(* Logix 5000 AddOnInstructionDefinition export AMP_Relative_Move; software revision 20.04 *)

TYPE AMP_Status_Word :   // Applied Motion Input Assembly Status Word
STRUCT
   Enabled : BOOL;   // Motor Enabled (Motor Disabled if this bit = 0)
   Sampling : BOOL;   // Sampling (for Quick Tuner)
   Drive_Fault : BOOL;   // Drive Fault (check Alarm Code)
   In_Position : BOOL;   // In Position (motor is in position)
   Moving : BOOL;   // Moving (motor is moving)
   Jogging : BOOL;   // Jogging (currently in jog mode)
   Stopping : BOOL;   // Stopping (in the process of stopping from a stop command)
   Waiting : BOOL;   // Waiting (for an input; executing a WI command)
   Saving : BOOL;   // Saving (parameter data is being saved)
   Alarm_Present : BOOL;   // Alarm present (check Alarm Code)
   Homing : BOOL;   // Homing (executing an SH command)
   Wait_Time : BOOL;   // Waiting (for time; executing a WD or WT command)
   Wizard_Running : BOOL;   // Wizard running (Timing Wizard is running)
   Checking_Encoder : BOOL;   // Checking encoder (Timing Wizard is running)
   Q_Program_Running : BOOL;   // Q Program is running
   Initializing : BOOL;   // Initializing (happens at power up) ; Servo Ready (for SV200 drives only)
END_STRUCT
END_TYPE

TYPE AMP_Alarm_Word :   // Applied Motion Input Assembly - Alarm Word
STRUCT
   Position_Limit : BOOL;   // Position Limit
   CCW_Limit : BOOL;   // CCW Limit
   CW_Limit : BOOL;   // CW Limit
   Over_Temp : BOOL;   // Over Temp
   Excess_Regen_or_Internal_Voltage : BOOL;   // Excess Regen or Internal Voltage
   Over_Voltage : BOOL;   // Over Voltage
   Under_Voltage : BOOL;   // Under Voltage
   Over_Current : BOOL;   // Over Current
   Open_Motor_Windings : BOOL;   // Open Motor Windings
   Bad_Encoder : BOOL;   // Bad Encoder
   Comm_Error : BOOL;   // Comm Error
   Bad_Flash : BOOL;   // Bad Flash
   No_Move : BOOL;   // No Move
   NA_1 : BOOL;   // NA 1
   Blank_Q_Segment : BOOL;   // Blank Q Segment
   NA_2 : BOOL;   // NA 2
END_STRUCT
END_TYPE

TYPE AMP_Input_Assembly_v2 :   // Applied Motion Drive Input Assembly Version 2.0
STRUCT
   Status_Code : DINT;   // Status Code
   Alarm_Code : DINT;   // Alarm Code
   Voltage : DINT;   // Supply Voltage (x0.1V)
   Current : DINT;   // Actual Current (mA)
   Temp : DINT;   // Drive Temperature (0.1 deg C)
   Encoder_Position : DINT;   // Encoder Position (20,000 counts = 1 shaft turn)
   Absolute_Position : DINT;   // Absolute Position (20,000 counts = 1 shaft turn)
   Position_Error : DINT;   // Position Error (counts)
   Actual_Velocity : DINT;   // Actual Velocity (rev/sec * 240, 0 when no encoder)
   Extended_Inputs : DINT;   // Input Status (Extended)
   Main_Board_Inputs : DINT;   // Input Status (Main board)
   Word11 : DINT;   // Reserved
   Analog_Input_1 : DINT;   // Analog Input 1 (ADC counts, 0=min V, 16383 = max V)
   Analog_Input_2 : DINT;   // Analog Input 2 (ADC counts, 0=min V, 16383 = max V)
END_STRUCT
END_TYPE

ADD_ON_INSTRUCTION AMP_Relative_Move   (* revision 1.0 *)
// Applied Motion - Relative Move AOI
// Help:
// The Relative Move AOI is used to move an axis by a specified distance (positive or negative) relative to its currently commanded position.
VAR_IN_OUT
   Input : DINT[14]; {required}   // Drive Input Assembly
   Output : DINT[16]; {required}   // Drive Output Assembly
        [0]   // Command Word
        [1]   // Jog Speed (0.25 rev/min)
        [2]   // Jog Acceleration (10 rev/s/s)
        [3]   // Jog Deceleration (10 rev/s/s)
        [4]   // Point-to-Point Velocity (0.25 rev/min)
        [5]   // Point-to-Point Acceleration (10 rev/min/s)
        [6]   // Point-to-Point Deceleration (10 rev/min/s)
        [7]   // Point-to-Point Distance (Motor steps)
        [9]   // (2x ASCII Letters in 16 lower word)
        [10]   // Data/Register 1
        [11]   // Data/Register 2
END_VAR
VAR_INPUT
   RPI : DINT := 100; {visible}   // Drive Connection Request Packet Interval (milliseconds)
   Start : BOOL; {required}   // Start the Relative Move
   Distance : DINT; {required}   // Relative Distance to Move (steps, negative = reverse)
   Speed : REAL; {required}   // Velocity of Move (rev/min)
   Acc : REAL; {required}   // Acceleration of Move (rev/s/s)
   Dec : REAL; {required}   // Deceleration (rev/s/s)
END_VAR
VAR_OUTPUT
   Sent : BOOL; {access Read Only, visible}   // Move has been sent to drive
   In_Progress : BOOL; {access Read Only, visible}   // Move in progress
   Done : BOOL; {access Read Only, visible}   // Move completed without errors - desired position reached
   Error : BOOL; {access Read Only, visible}   // Move failed to complete - drive not ready or faulted
   State : DINT := 10; {access Read Only}   // Internal state of progress
END_VAR
VAR
   Loc_StatusCode : AMP_Status_Word;
   Loc_CommandOff_Timer : TIMER;   // Timer to make sure command value was 0 before sending a new command
   Loc_CommandOn_Timer : TIMER;   // Timer to make sure command value is set long enough to be sent to drive
   Loc_Input_Assembly : AMP_Input_Assembly_v2; {access None}
   Loc_Start_ONS : BOOL; {access None}
   Loc_AlarmCode : AMP_Alarm_Word; {access None}
END_VAR

ROUTINE Logic   (* ladder *)
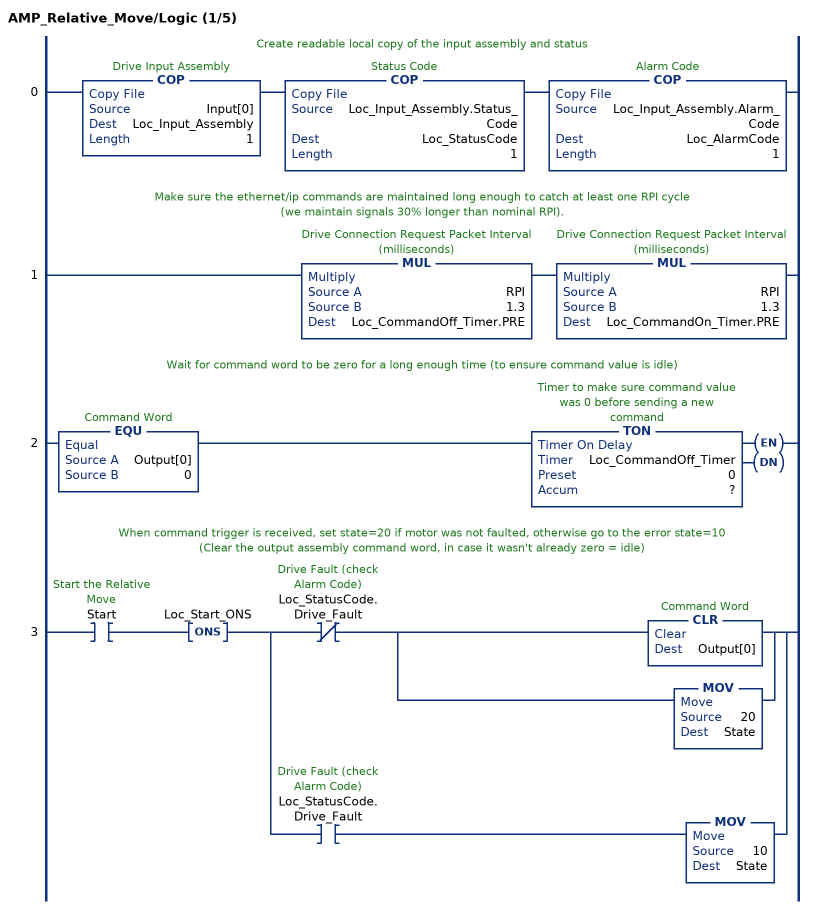
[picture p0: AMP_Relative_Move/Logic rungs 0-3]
   // Create readable local copy of the input assembly and status
   0: COP(Input[0],Loc_Input_Assembly,1)COP(Loc_Input_Assembly.Status_Code,Loc_StatusCode,1)COP(Loc_Input_Assembly.Alarm_Code,Loc_AlarmCode,1);
   // Make sure the ethernet/ip commands are maintained long enough to catch at least one RPI cycle
   // (we maintain signals 30% longer than nominal RPI).
   1: MUL(RPI,1.3,Loc_CommandOff_Timer.PRE)MUL(RPI,1.3,Loc_CommandOn_Timer.PRE);
   // Wait for command word to be zero for a long enough time (to ensure command value is idle)
   2: EQU(Output[0],0)TON(Loc_CommandOff_Timer,?,?);
   // When command trigger is received, set state=20 if motor was not faulted, otherwise go to the error state=10
   // (Clear the output assembly command word, in case it wasn't already zero = idle)
   3: XIC(Start)ONS(Loc_Start_ONS)[XIO(Loc_StatusCode.Drive_Fault) [CLR(Output[0]) ,MOV(20,State) ] ,XIC(Loc_StatusCode.Drive_Fault) MOV(10,State) ];
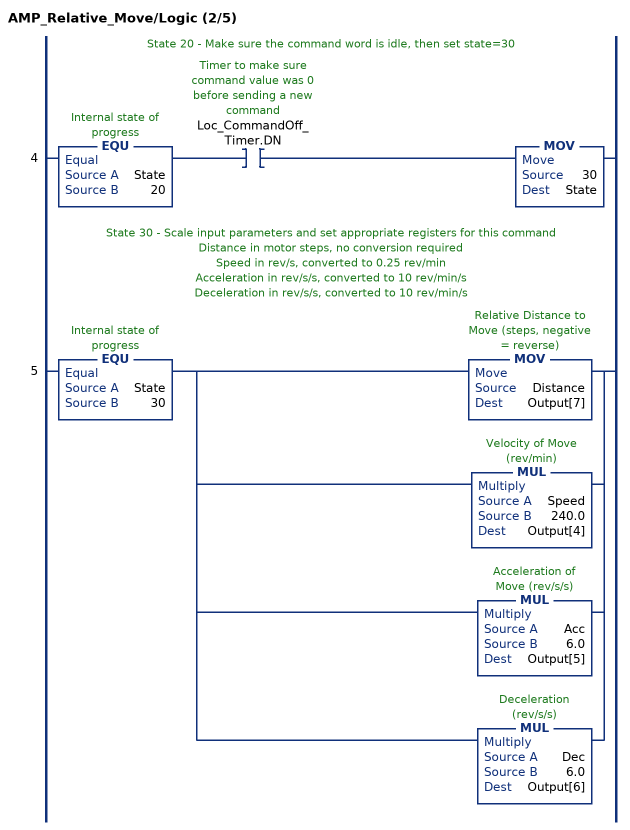
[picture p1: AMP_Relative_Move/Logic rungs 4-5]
   // State 20 - Make sure the command word is idle, then set state=30
   4: EQU(State,20)XIC(Loc_CommandOff_Timer.DN)MOV(30,State);
   // State 30 - Scale input parameters and set appropriate registers for this command
   // Distance in motor steps, no conversion required
   // Speed in rev/s, converted to 0.25 rev/min
   // Acceleration in rev/s/s, converted to 10 rev/min/s
   // Deceleration in rev/s/s, converted to 10 rev/min/s
   5: EQU(State,30)[MOV(Distance,Output[7]) ,MUL(Speed,240.0,Output[4]) ,MUL(Acc,6.0,Output[5]) ,MUL(Dec,6.0,Output[6]) ];
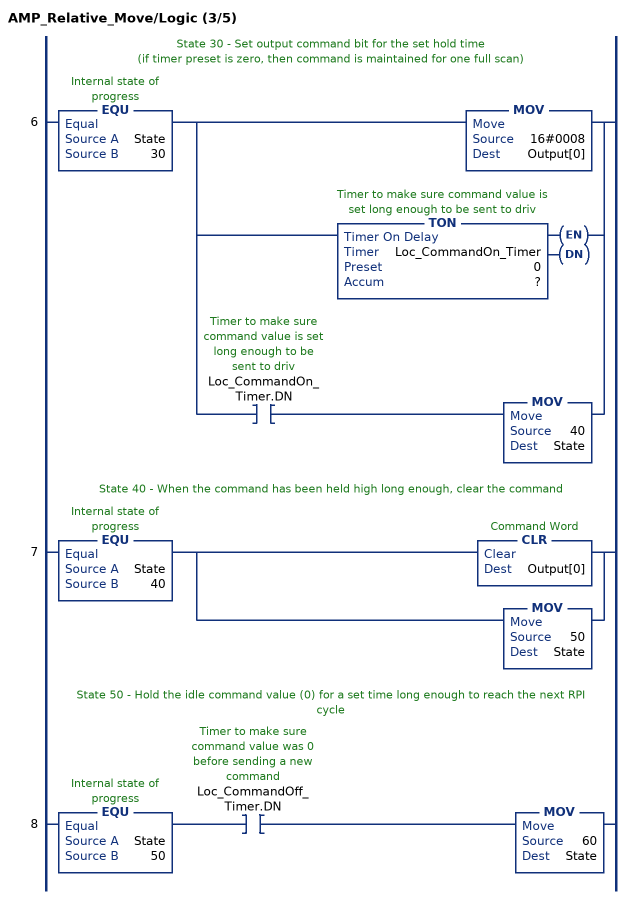
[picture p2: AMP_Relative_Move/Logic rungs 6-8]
   // State 30 - Set output command bit for the set hold time
   // (if timer preset is zero, then command is maintained for one full scan)
   6: EQU(State,30)[MOV(16#0008,Output[0]) ,TON(Loc_CommandOn_Timer,?,?) ,XIC(Loc_CommandOn_Timer.DN) MOV(40,State) ];
   // State 40 - When the command has been held high long enough, clear the command
   7: EQU(State,40)[CLR(Output[0]) ,MOV(50,State) ];
   // State 50 - Hold the idle command value (0) for a set time long enough to reach the next RPI cycle
   8: EQU(State,50)XIC(Loc_CommandOff_Timer.DN)MOV(60,State);
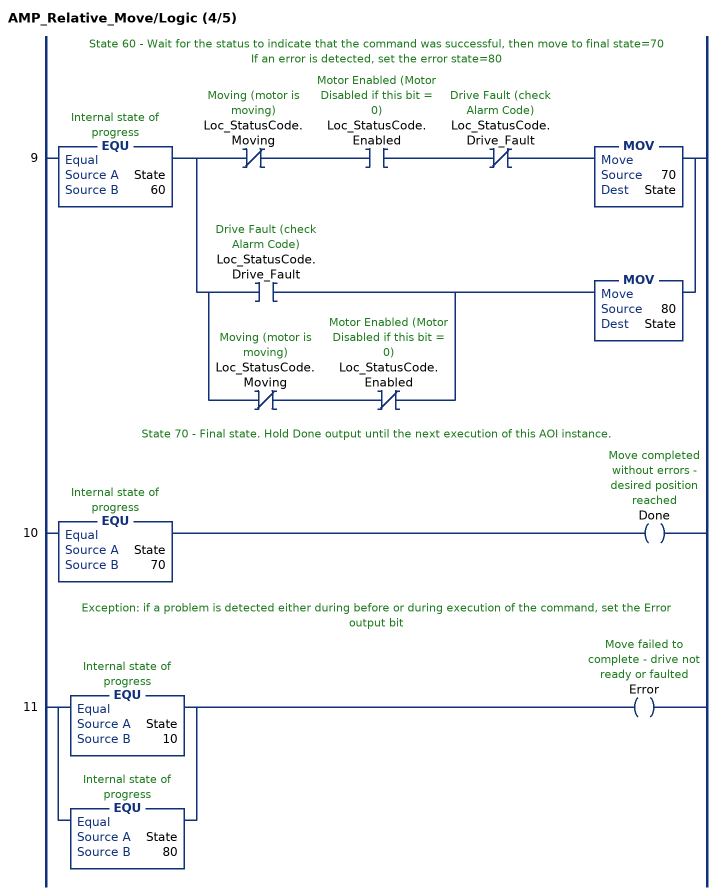
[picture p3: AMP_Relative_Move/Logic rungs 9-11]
   // State 60 - Wait for the status to indicate that the command was successful, then move to final state=70
   // If an error is detected, set the error state=80
   9: EQU(State,60)[XIO(Loc_StatusCode.Moving) XIC(Loc_StatusCode.Enabled) XIO(Loc_StatusCode.Drive_Fault) MOV(70,State) ,[XIC(Loc_StatusCode.Drive_Fault) ,XIO(Loc_StatusCode.Moving) XIO(Loc_StatusCode.Enabled) ] MOV(80,State) ];
   // State 70 - Final state. Hold Done output until the next execution of this AOI instance.
   10: EQU(State,70)OTE(Done);
   // Exception: if a problem is detected either during before or during execution of the command, set the Error output bit
   11: [EQU(State,10) ,EQU(State,80) ]OTE(Error);
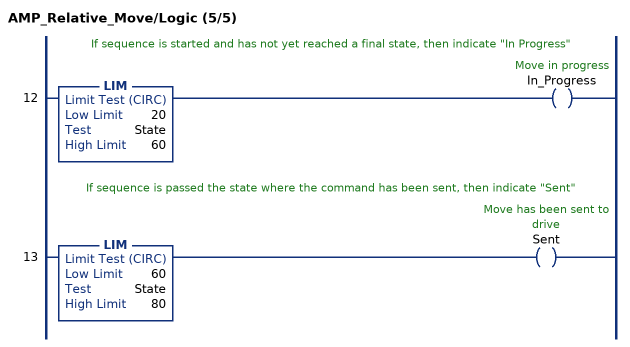
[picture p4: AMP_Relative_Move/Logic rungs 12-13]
   // If sequence is started and has not yet reached a final state, then indicate "In Progress"
   12: LIM(20,State,60)OTE(In_Progress);
   // If sequence is passed the state where the command has been sent, then indicate "Sent"
   13: LIM(60,State,80)OTE(Sent);
END_ROUTINE
END_ADD_ON_INSTRUCTION
